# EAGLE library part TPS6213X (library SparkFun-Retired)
3-17V, 3A Step Down Converter(new? IC-11155)
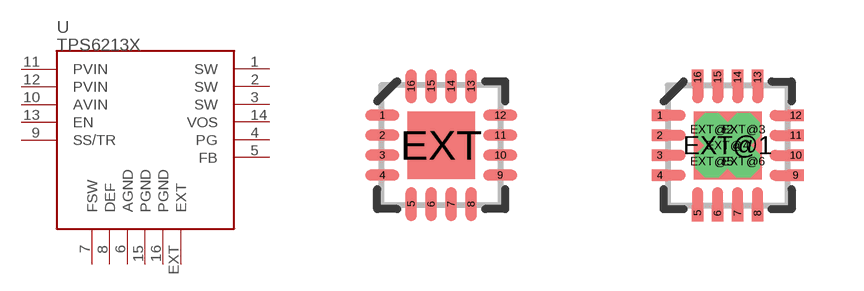
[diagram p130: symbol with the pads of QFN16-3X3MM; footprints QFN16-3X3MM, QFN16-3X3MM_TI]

Designator prefix -

## TPS6213XV1 (PROD_ID: IC-11630)  [QFN16-3X3MM]
1  SW
2  SW
3  SW
4  PG
5  FB
6  AGND
7  FSW
8  DEF
9  SS/TR
10  AVIN
11  PVIN
12  PVIN
13  EN
14  VOS
15  PGND
16  PGND
EXT  EXT

## TPS6213XTI  [QFN16-3X3MM_TI]
1  SW
2  SW
3  SW
4  PG
5  FB
6  AGND
7  FSW
8  DEF
9  SS/TR
10  AVIN
11  PVIN
12  PVIN
13  EN
14  VOS
15  PGND
16  PGND
EXT@1  EXT
EXT@2  EXT
EXT@3  EXT
EXT@4  EXT
EXT@5  EXT
EXT@6  EXT

## Footprint QFN16-3X3MM (pad centres in mm)
3mm x 3mm QFN 16 pin
smd 0.85 x 0.28: 1 -1.475,0.75; 2 -1.475,0.25; 3 -1.475,-0.25; 4 -1.475,-0.75; 9 1.475,-0.75; 10 1.475,-0.25; 11 1.475,0.25; 12 1.475,0.75
smd 0.28 x 0.85: 5 -0.75,-1.475; 6 -0.25,-1.475; 7 0.25,-1.475; 8 0.75,-1.475; 13 0.75,1.475; 14 0.25,1.475; 15 -0.25,1.475; 16 -0.75,1.475
smd 1.68 x 1.68: EXT 0,0

## Footprint QFN16-3X3MM_TI (pad centres in mm)
smd 0.4 x 0.28: 1 -1.7,0.75; 2 -1.7,0.25; 3 -1.7,-0.25; 4 -1.7,-0.75; 9 1.7,-0.75; 10 1.7,-0.25; 11 1.7,0.25; 12 1.7,0.75
smd 0.28 x 0.4: 5 -0.75,-1.7; 6 -0.25,-1.7; 7 0.25,-1.7; 8 0.75,-1.7; 13 0.75,1.7; 14 0.25,1.7; 15 -0.25,1.7; 16 -0.75,1.7
smd 1.7 x 1.7: EXT@1 0,0
drill 0.3 octagon: EXT@2 -0.4,0.4; EXT@3 0.4,0.4; EXT@4 0,0; EXT@5 -0.4,-0.4; EXT@6 0.4,-0.4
